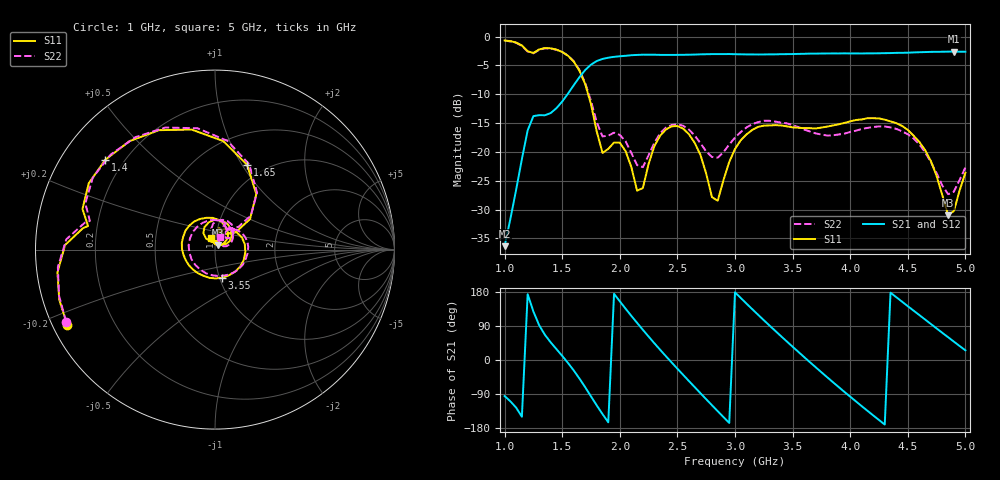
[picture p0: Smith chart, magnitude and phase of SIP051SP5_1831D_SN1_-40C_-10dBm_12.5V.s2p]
# GHz  S  dB  R  50
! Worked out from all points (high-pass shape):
!   81 points, 1 GHz to 5 GHz, reference 50 ohm
!   highest |S21| = -2.62 dB at 4.9 GHz (marker M1); lowest = -36.4 dB at 1 GHz (marker M2)
!   |S21| within 3 dB of the highest: 1.71 GHz to end of sweep
!   lowest |S11| = -31.0 dB at 4.85 GHz (marker M3), VSWR 1.06, Z = 51.6 + j2.38 ohm
!   |S11| at or under -10 dB: 1.725 GHz to end of sweep
!   |S22| runs from -27.3 to -0.7 dB; largest |S21 - S12| = 0.0021
!   S11 on the Smith chart (normalised r, x): 1 GHz: 0.04, -0.24; 1.4 GHz: 0.13, +0.35; 1.65 GHz: 0.83, +1.05; 3.55 GHz: 1.03, -0.33; 5 GHz: 0.95, +0.12
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1  -0.69 -153.1  -36.35 -95.2  -36.20 -94.8  -0.71 -154.2
1.2  -2.56 170.7  -16.27 173.6  -16.28 173.8  -2.61 168.3
1.4  -2.05 140.6  -13.28 46.6  -13.26 46.7  -2.09 137.7
1.65  -5.94 69.3  -7.04 -49.2  -7.04 -49.1  -5.82 68.1
1.7  -8.27 53.4  -5.80 -72.2  -5.81 -72.1  -8.08 53.5
1.85  -20.19 61.1  -3.89 -142.8  -3.88 -142.7  -17.32 58.3
1.95  -18.39 80.4  -3.52 174.7  -3.54 174.8  -16.68 69.7
2.15  -26.74 77.2  -3.19 98.0  -3.20 98.1  -22.29 67.2
2.35  -17.20 115.3  -3.19 27.0  -3.16 27.0  -16.77 94.1
2.5  -15.52 76.9  -3.19 -23.0  -3.19 -23.0  -15.23 65.9
2.7  -20.52 29.7  -3.09 -87.6  -3.08 -87.5  -18.50 38.2
2.85  -28.47 74.0  -3.05 -135.1  -3.04 -135.1  -21.00 53.7
3  -19.50 76.4  -3.07 178.6  -3.06 178.6  -17.54 56.5
3.3  -15.42 -4.4  -3.09 90.9  -3.10 90.9  -14.62 4.8
3.55  -15.82 -76.0  -3.02 21.4  -3.00 21.3  -15.70 -52.6
3.7  -15.94 -114.3  -2.97 -19.0  -2.96 -19.1  -16.81 -94.8
4  -14.71 178.9  -2.94 -96.8  -2.94 -96.8  -16.55 171.0
4.35  -14.71 105.2  -2.87 177.6  -2.88 177.7  -15.76 80.7
4.6  -18.27 54.5  -2.73 118.6  -2.73 118.6  -18.70 31.2
4.85  -30.97 54.5  -2.62 60.1  -2.63 60.2  -27.34 36.5
4.9  -30.26 89.5  -2.62 48.5  -2.63 48.5  -26.90 55.1
5  -23.64 108.3  -2.64 25.5  -2.64 25.4  -22.70 69.1
